FUNCTION_BLOCK Example08_bufferstatus //4x3 flyways 2 xbots - get pmc state, get buffer status
VAR_INPUT
	Execute : BOOL;
END_VAR
VAR_OUTPUT
	Done : BOOL;
END_VAR
VAR_IN_OUT
	PM_Controller : PMControllerType;	// the planar motor controller to use
END_VAR
VAR
	pmc_state1 : USINT;
	nxbots1 : UINT;
	PMC_GetPmcStatus1 : PMC_GetPmcStatus;
	buffer_state1 : USINT;
	ncmds1 : UINT;
	PMC_GetBufferStatus1 : PMC_GetBufferStatus;
	PMC_MotionBufferCtrl1 : PMC_MotionBufferCtrl;
	buffer_state2 : USINT;
	ncmds2 : UINT;
	PMC_GetBufferStatus2 : PMC_GetBufferStatus;
	PMC_XYMotion1 : PMC_XYMotion;
	PMC_XYMotion2 : PMC_XYMotion;
	buffer_state3 : USINT;
	ncmds3 : UINT;
	PMC_GetBufferStatus3 : PMC_GetBufferStatus;
	PMC_MotionBufferCtrl2 : PMC_MotionBufferCtrl;
END_VAR

//4x3 flyways 2 xbots - get pmc state, get buffer status

//get pmc state
PMC_GetPmcStatus1(Execute := Execute,State => pmc_state1,nXbots => nxbots1,PM_Controller := PM_Controller);

//get buffer status of xbot 1
PMC_GetBufferStatus1(Execute := PMC_GetPmcStatus1.Valid,XbotID := 1,State => buffer_state1,nCmds => ncmds1,PM_Controller := PM_Controller);

//block buffer of xbot 1
PMC_MotionBufferCtrl1(Execute := PMC_GetBufferStatus1.Valid,Level := 0,XbotID := 1,PM_Controller := PM_Controller);

//get buffer status of xbot 1
PMC_GetBufferStatus2(Execute := PMC_MotionBufferCtrl1.Done,XbotID := 1,State => buffer_state2,nCmds => ncmds2,PM_Controller := PM_Controller);

//add move command to xbot 1 buffer
PMC_XYMotion1(Execute := PMC_GetBufferStatus2.Valid,cmdLB := 5,XbotID := 1,Mode := 0,Type_ := 0,PosX := 0.9,PosY := 0.06,EndVel := 0,MaxVel := 1,MaxAcc := 10,PM_Controller := PM_Controller);

//add move command to xbot 1 buffer
PMC_XYMotion2(Execute := PMC_XYMotion1.Ack,cmdLB := 6,XbotID := 1,Mode := 0,Type_ := 0,PosX := 0.06,PosY := 0.06,EndVel := 0,MaxVel := 1,MaxAcc := 10,PM_Controller := PM_Controller);

//get buffer status of xbot 1
PMC_GetBufferStatus3(Execute := PMC_XYMotion2.Ack,XbotID := 1,State => buffer_state3,nCmds => ncmds3,PM_Controller := PM_Controller);

//release buffer of xbot 1
PMC_MotionBufferCtrl2(Execute := PMC_GetBufferStatus3.Valid,Level := 1,XbotID := 1,PM_Controller := PM_Controller);

Done := PMC_XYMotion2.Done;

END_FUNCTION_BLOCK
